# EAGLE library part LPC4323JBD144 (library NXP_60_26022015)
32-bit ARM Cortex-M4/M0 MCU; up to 1 MB flash and 136 kB SRAM; Ethernet, two High-speed USB, LCD, EMC The LPC435x/3x/2x/1x are ARM Cortex-M4 based microcontrollers for embedded applications which include an ARM Cortex-M0 coprocessor, up to 1 MB of flash and 136 kB of on-chip SRAM, 16 kB of EEPROM memory, a quad SPI Flash Interface (SPIFI), advanced configurable peripherals such as the State Configurable Timer (SCT) and the Serial General Purpose I/O (SGPIO) interface, two High-speed USB controllers, Ethernet, LCD, an external memory controller, and multiple digital and analog peripherals. The LPC435x/3x/2x/1x operate at CPU frequencies of up to 204 MHz. The ARM Cortex-M4 is a next generation 32-bit core that offers system enhancements such as low power consumption, enhanced debug features, and a high level of support block integration. The ARM Cortex-M4 CPU incorporates a 3-stage pipeline, uses a Harvard architecture with separate local instruction and data buses as well as a third bus for peripherals, and includes an internal prefetch unit that supports speculative branching. The ARM Cortex-M4 supports single-cycle digital signal processing and SIMD instructions. A hardware floating-point unit is integrated in the core. The ARM Cortex-M0 coprocessor is an energy-efficient and easy-to-use 32-bit core which is upward code- and tool-compatible with the Cortex-M4 core. The Cortex-M0 coprocessor, designed as a replacement for existing 8/16-bit microcontrollers, offers up to 204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
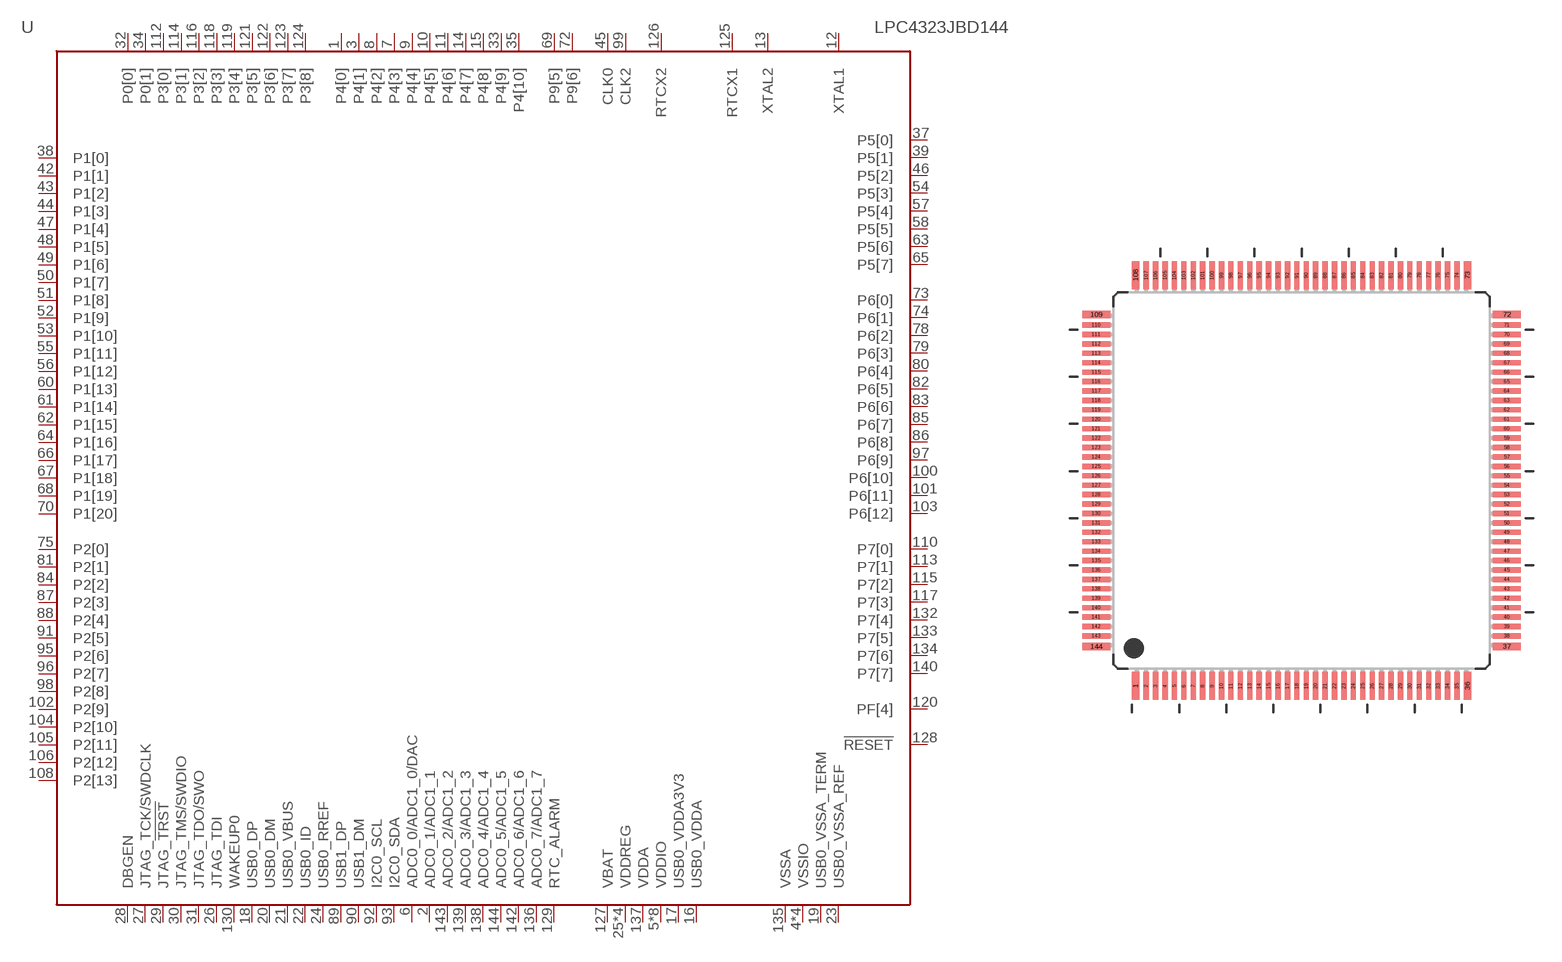
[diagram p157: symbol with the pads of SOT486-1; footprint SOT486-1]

Designator prefix U

## LPC4323JBD144  [SOT486-1]
1  P4[0]
2  ADC0_1/ADC1_1  in
3  P4[1]
4  VSSIO  pwr
5  VDDIO  pwr
6  ADC0_0/ADC1_0/DAC  in
7  P4[3]
8  P4[2]
9  P4[4]
10  P4[5]
11  P4[6]
12  XTAL1  in
13  XTAL2  out
14  P4[7]
15  P4[8]
16  USB0_VDDA  pwr
17  USB0_VDDA3V3  pwr
18  USB0_DP
19  USB0_VSSA_TERM  pwr
20  USB0_DM
21  USB0_VBUS
22  USB0_ID  in
23  USB0_VSSA_REF  pwr
24  USB0_RREF  pas
25  VDDREG  pwr
26  JTAG_TDI  in
27  JTAG_TCK/SWDCLK  in
28  DBGEN  in
29  JTAG_!TRST  in
30  JTAG_TMS/SWDIO  in
31  JTAG_TDO/SWO  out
32  P0[0]
33  P4[9]
34  P0[1]
35  P4[10]
36  VDDIO  pwr
37  P5[0]
38  P1[0]
39  P5[1]
40  VSSIO  pwr
41  VDDIO  pwr
42  P1[1]
43  P1[2]
44  P1[3]
45  CLK0
46  P5[2]
47  P1[4]
48  P1[5]
49  P1[6]
50  P1[7]
51  P1[8]
52  P1[9]
53  P1[10]
54  P5[3]
55  P1[11]
56  P1[12]
57  P5[4]
58  P5[5]
59  VDDREG  pwr
60  P1[13]
61  P1[14]
62  P1[15]
63  P5[6]
64  P1[16]
65  P5[7]
66  P1[17]
67  P1[18]
68  P1[19]
69  P9[5]
70  P1[20]
71  VDDIO  pwr
72  P9[6]
73  P6[0]
74  P6[1]
75  P2[0]
76  VSSIO  pwr
77  VDDIO  pwr
78  P6[2]
79  P6[3]
80  P6[4]
81  P2[1]
82  P6[5]
83  P6[6]
84  P2[2]
85  P6[7]
86  P6[8]
87  P2[3]
88  P2[4]
89  USB1_DP
90  USB1_DM
91  P2[5]
92  I2C0_SCL
93  I2C0_SDA
94  VDDREG  pwr
95  P2[6]
96  P2[7]
97  P6[9]
98  P2[8]
99  CLK2
100  P6[10]
101  P6[11]
102  P2[9]
103  P6[12]
104  P2[10]
105  P2[11]
106  P2[12]
107  VDDIO  pwr
108  P2[13]
109  VSSIO  pwr
110  P7[0]
111  VDDIO  pwr
112  P3[0]
113  P7[1]
114  P3[1]
115  P7[2]
116  P3[2]
117  P7[3]
118  P3[3]
119  P3[4]
120  PF[4]
121  P3[5]
122  P3[6]
123  P3[7]
124  P3[8]
125  RTCX1  in
126  RTCX2  out
127  VBAT  pwr
128  !RESET!  in
129  RTC_ALARM  out
130  WAKEUP0  in
131  VDDREG  pwr
132  P7[4]
133  P7[5]
134  P7[6]
135  VSSA  pwr
136  ADC0_7/ADC1_7  in
137  VDDA  pwr
138  ADC0_4/ADC1_4  in
139  ADC0_3/ADC1_3  in
140  P7[7]
141  VDDIO  pwr
142  ADC0_6/ADC1_6  in
143  ADC0_2/ADC1_2  in
144  ADC0_5/ADC1_5  in

## Footprint SOT486-1 (pad centres in mm)
SOT486-1 LQFP144: plastic low profile quad flat package; 144 leads; body 20 x 20 x 1.4 mm JEDEC: MS-026 IEC: 136E23
smd 0.4 x 1.5: 1 -8.81,-10.9; 36 8.81,-10.9; 73 8.81,10.9; 108 -8.81,10.9
smd 0.28 x 1.5: 2 -8.25,-10.9; 3 -7.75,-10.9; 4 -7.25,-10.9; 5 -6.75,-10.9; 6 -6.25,-10.9; 7 -5.75,-10.9; 8 -5.25,-10.9; 9 -4.75,-10.9; 10 -4.25,-10.9; 11 -3.75,-10.9; 12 -3.25,-10.9; 13 -2.75,-10.9; 14 -2.25,-10.9; 15 -1.75,-10.9; 16 -1.25,-10.9; 17 -0.75,-10.9; 18 -0.25,-10.9; 19 0.25,-10.9; 20 0.75,-10.9; 21 1.25,-10.9; 22 1.75,-10.9; 23 2.25,-10.9; 24 2.75,-10.9; 25 3.25,-10.9; 26 3.75,-10.9; 27 4.25,-10.9; 28 4.75,-10.9; 29 5.25,-10.9; 30 5.75,-10.9; 31 6.25,-10.9; 32 6.75,-10.9; 33 7.25,-10.9; 34 7.75,-10.9; 35 8.25,-10.9; 74 8.25,10.9; 75 7.75,10.9; 76 7.25,10.9; 77 6.75,10.9; 78 6.25,10.9; 79 5.75,10.9; 80 5.25,10.9; 81 4.75,10.9; 82 4.25,10.9; 83 3.75,10.9; 84 3.25,10.9; 85 2.75,10.9; 86 2.25,10.9; 87 1.75,10.9; 88 1.25,10.9; 89 0.75,10.9; 90 0.25,10.9; 91 -0.25,10.9; 92 -0.75,10.9; 93 -1.25,10.9; 94 -1.75,10.9; 95 -2.25,10.9; 96 -2.75,10.9; 97 -3.25,10.9; 98 -3.75,10.9; 99 -4.25,10.9; 100 -4.75,10.9; 101 -5.25,10.9; 102 -5.75,10.9; 103 -6.25,10.9; 104 -6.75,10.9; 105 -7.25,10.9; 106 -7.75,10.9; 107 -8.25,10.9
smd 1.5 x 0.4: 37 10.9,-8.81; 72 10.9,8.81; 109 -10.9,8.81; 144 -10.9,-8.81
smd 1.5 x 0.28: 38 10.9,-8.25; 39 10.9,-7.75; 40 10.9,-7.25; 41 10.9,-6.75; 42 10.9,-6.25; 43 10.9,-5.75; 44 10.9,-5.25; 45 10.9,-4.75; 46 10.9,-4.25; 47 10.9,-3.75; 48 10.9,-3.25; 49 10.9,-2.75; 50 10.9,-2.25; 51 10.9,-1.75; 52 10.9,-1.25; 53 10.9,-0.75; 54 10.9,-0.25; 55 10.9,0.25; 56 10.9,0.75; 57 10.9,1.25; 58 10.9,1.75; 59 10.9,2.25; 60 10.9,2.75; 61 10.9,3.25; 62 10.9,3.75; 63 10.9,4.25; 64 10.9,4.75; 65 10.9,5.25; 66 10.9,5.75; 67 10.9,6.25; 68 10.9,6.75; 69 10.9,7.25; 70 10.9,7.75; 71 10.9,8.25; 110 -10.9,8.25; 111 -10.9,7.75; 112 -10.9,7.25; 113 -10.9,6.75; 114 -10.9,6.25; 115 -10.9,5.75; 116 -10.9,5.25; 117 -10.9,4.75; 118 -10.9,4.25; 119 -10.9,3.75; 120 -10.9,3.25; 121 -10.9,2.75; 122 -10.9,2.25; 123 -10.9,1.75; 124 -10.9,1.25; 125 -10.9,0.75; 126 -10.9,0.25; 127 -10.9,-0.25; 128 -10.9,-0.75; 129 -10.9,-1.25; 130 -10.9,-1.75; 131 -10.9,-2.25; 132 -10.9,-2.75; 133 -10.9,-3.25; 134 -10.9,-3.75; 135 -10.9,-4.25; 136 -10.9,-4.75; 137 -10.9,-5.25; 138 -10.9,-5.75; 139 -10.9,-6.25; 140 -10.9,-6.75; 141 -10.9,-7.25; 142 -10.9,-7.75; 143 -10.9,-8.25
